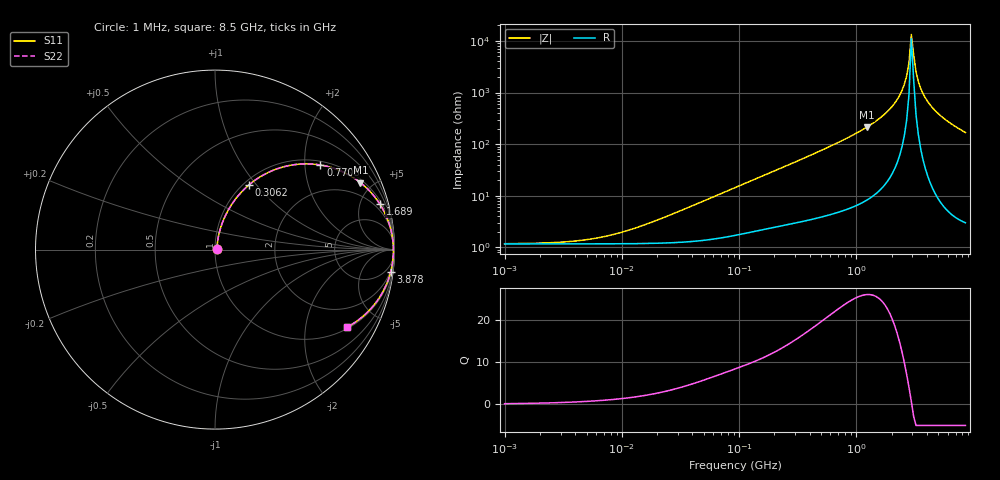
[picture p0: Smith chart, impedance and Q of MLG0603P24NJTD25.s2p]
! S-Parameter Data Generated by TDK Corporation
! Copyright(C) 2025 TDK Corporation.
! All Rights Reserved.
! TDK P/N: MLG0603P24NJTD25 (SMD / SMT Inductor (Coil))
! Property: L=24nH at 500MHz
! Size(LxWxT): 0.6x0.3x0.3mm
! Model Type: s2p (Touchstone File Format Version 1.0)
! Frequency: DC=Yes Start=1MHz Stop=8500MHz 198points Log-sweep
! Model Generated on Feb. 6, 2025
! Terms and conditions regarding TDK Simulation Models:
! 1)This simulation model is being provided solely for informational
!  purposes. Please refer to the specifications of the products in
!  terms of detailed characteristics of such products.
! 2)In no event shall TDK Corporation of any of its subsidiaries be
!  liable for any loss or damage arising, directly or indirectly,
!  from any information contained in this simulation model, including,
!  but not limited to loss or damages arising from any inaccuracies,
!  omissions or errors in connection with such information.
! 3)Any and all copyrights on this simulation model are owned by
!  TDK Corporation.  Duplication or redistribution of this simulation
!  model without prior written permission from TDK Corporation
!  is prohibited.
! 4)This simulation model is subject to any modification or change
!  without any prior notice.
! 5)Neither TDK Corporation nor any of its subsidiaries shall make any
!  warranty, express or implied, including but not limited to the
!  correctness, implied warranties of merchantability and fitness for
!  a particular purpose with respect to this simulation models.
! 6)The use of this simulation model shall be deemed to have consented
!  to the terms and conditions hereof.
! Port Assignments:
!  1 ---@@@--- 2
! Applicable Conditions:
!  Temperature = 25 degC
!  DC Bias Current = 0 A
!  Small Signal Operation
# Hz S MA R 50
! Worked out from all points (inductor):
!   197 points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, 1 MHz to 8.5 GHz, reference 50 ohm
!   read as one part in series: L = 25.1 nH near 24.17 MHz
!   highest Q = 25.9 at 1.223 GHz (marker M1), where L = 27.7 nH
!   self-resonance near 2.94 GHz
!   S11 on the Smith chart (normalised r, x): 1 MHz: 1.02, +0.00; 306.2 MHz: 1.06, +0.92; 770.8 MHz: 1.10, +2.40; 1.689 GHz: 1.30, +7.19; 3.878 GHz: 2, -16; 8.5 GHz: 1.06, -3.37
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1000000  0.01167 7.6  0.9884 -0.1  0.9884 -0.1  0.01167 7.6
4587603  0.01363 31.4  0.9884 -0.4  0.9884 -0.4  0.01363 31.4
9601846  0.019 51.3  0.9882 -0.9  0.9882 -0.9  0.019 51.3
2.10461e7  0.03495 68.1  0.9875 -1.9  0.9875 -1.9  0.03495 68.1
9.219544e7  0.1398 75.2  0.9736 -8.0  0.9736 -8.0  0.1398 75.2
1.842597e8  0.2636 69.9  0.9426 -15.2  0.9426 -15.2  0.2636 69.9
3.061674e8  0.4078 62.3  0.8869 -24.0  0.8869 -24.0  0.4078 62.3
4.229561e8  0.5236 55.3  0.8235 -31.5  0.8235 -31.5  0.5236 55.3
7.707615e8  0.7531 38.7  0.6265 -48.8  0.6265 -48.8  0.7531 38.7
1.222927e9  0.8919 24.8  0.4191 -63.0  0.4191 -63.0  0.8919 24.8
1.689417e9  0.9533 15.4  0.265 -72.3  0.265 -72.3  0.9533 15.4
1.940355e9  0.9706 11.5  0.1992 -75.8  0.1992 -75.8  0.9706 11.5
2.333852e9  0.9861 6.4  0.1123 -79.7  0.1123 -79.7  0.9861 6.4
2.559585e9  0.9907 3.9  0.06924 -80.3  0.06924 -80.3  0.9907 3.9
2.680511e9  0.9922 2.7  0.04778 -79.3  0.04778 -79.3  0.9922 2.7
2.80715e9  0.9933 1.5  0.02654 -74.6  0.02654 -74.6  0.9933 1.5
2.939772e9  0.9938 0.2  0.007458 -33.9  0.007458 -33.9  0.9938 0.2
3.224109e9  0.9934 -2.2  0.03945 79.3  0.03945 79.3  0.9934 -2.2
3.535948e9  0.9911 -4.7  0.08259 81.4  0.08259 81.4  0.9911 -4.7
3.877948e9  0.9867 -7.2  0.1262 80.3  0.1262 80.3  0.9867 -7.2
5.357206e9  0.9538 -16.4  0.2817 72.5  0.2817 72.5  0.9538 -16.4
8.5e9  0.8531 -30.4  0.5068 58.5  0.5068 58.5  0.8531 -30.4
